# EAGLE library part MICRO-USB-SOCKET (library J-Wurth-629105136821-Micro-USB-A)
WR-COM SMT Horizontal 5 Contacts Micro USB Type B,5 pins=>Code : Con_I-O_COM_MicroUSB_629105136821 Details see: http://katalog.we-online.de/en/em/COM_MICRO_SMT_TYPE_B_HORIZONTAL/629105136821?m Created 2014-07-09, Karrer Zheng 2014 (C) Würth Elektronik
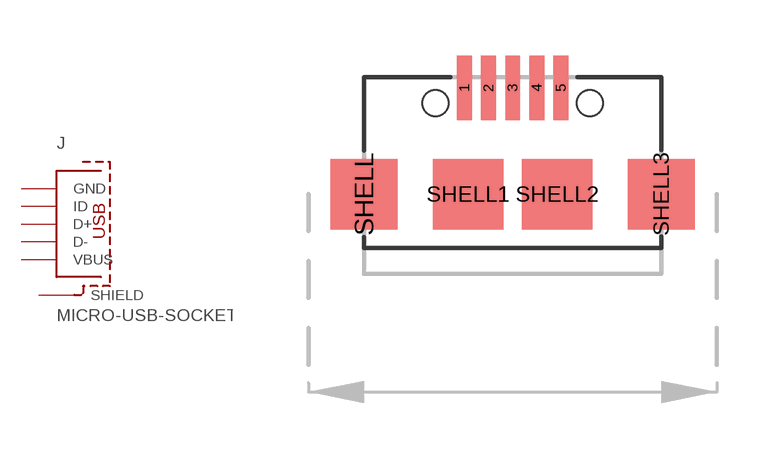
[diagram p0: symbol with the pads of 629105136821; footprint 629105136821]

Designator prefix J

## MICRO-USB-SOCKET  [629105136821]
1  VBUS  pas
2  D-  pas
3  D+  pas
4  ID  pas
5  GND  pas
SHELL  SHIELD  pas
SHELL1  SHIELD  pas
SHELL2  SHIELD  pas
SHELL3  SHIELD  pas

## Footprint 629105136821 (pad centres in mm)
WR-COM SMT Horizontal 5 Contacts Micro USB Type B, 5 pins
smd 0.4 x 1.731: 1 -1.3,2.865; 2 -0.65,2.865; 3 0,2.865; 4 0.65,2.865; 5 1.3,2.865
smd 1.8 x 1.9: SHELL -4,0; SHELL3 4,0
smd 1.9 x 1.9: SHELL1 -1.2,0; SHELL2 1.2,0
hole 0.7 at -2.075,2.45
hole 0.7 at 2.075,2.45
